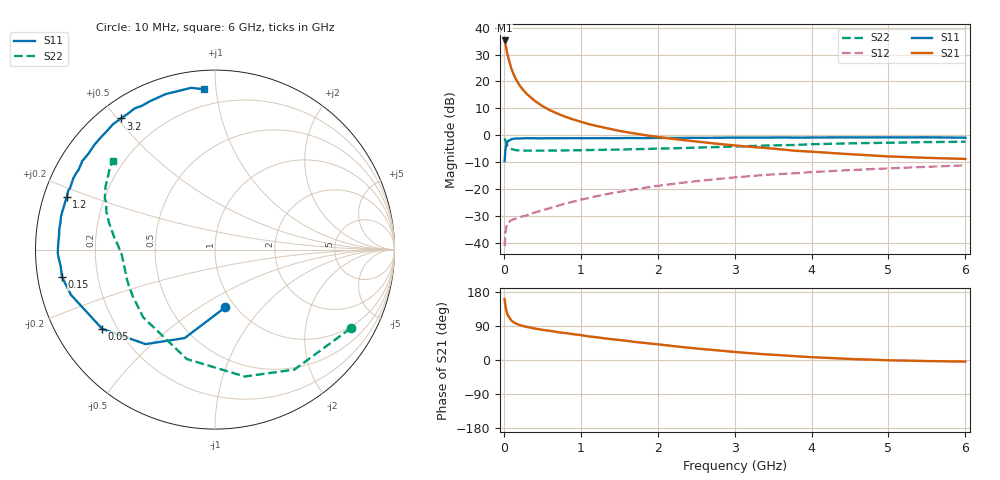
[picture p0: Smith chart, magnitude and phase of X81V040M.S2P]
! SIEMENS Small Signal Semiconductors
! BFP136W
! Si NPN RF Bipolar Junction Transistor in SOT343
! VCE = 1 V  IC = 40 mA
! Common Emitter S-Parameters:  September  1994
# GHz  S  MA  R  50
!  f  S11  S21  S12  S22
! GHz  MAG  ANG  MAG  ANG  MAG  ANG  MAG  ANG
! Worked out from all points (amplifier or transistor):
!   40 points, 10 MHz to 6 GHz, reference 50 ohm
!   highest |S21| = 35.2 dB at 10 MHz (marker M1)
!   |S21| within 3 dB of that: start of sweep to 32.17 MHz
!   unconditionally stable (mu >= 1): 616.7 MHz to 2.95 GHz; 3.767 GHz to 3.848 GHz; 5.876 GHz to end of sweep
!   at 200 MHz: K = 0.52, MSG = 24.6 dB, |S12| = -30.6 dB
!   at 1.5 GHz: K = 1.15, MAG = 9.0 dB, |S12| = -21.1 dB
!   at 6 GHz: K = 1.01, MAG = 0.5 dB, |S12| = -11.2 dB
!   S11 on the Smith chart (normalised r, x): 10 MHz: 0.90, -0.65; 50 MHz: 0.14, -0.31; 150 MHz: 0.07, -0.09; 1.2 GHz: 0.07, +0.17; 3.2 GHz: 0.07, +0.51; 6 GHz: 0.10, +0.93
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0.01  0.3272 -80.1  57.71 160.6  0.0086 69.3  0.874 -30.1
0.02  0.5209 -108.9  49.83 144.5  0.0151 55.6  0.8017 -56.5
0.03  0.6535 -126.3  42.35 132.8  0.0192 47.0  0.7262 -76.8
0.05  0.7679 -144.9  30.38 118.4  0.0234 34.8  0.6297 -104.4
0.1  0.8408 -162.5  16.84 103.5  0.0262 27.7  0.55 -136.7
0.15  0.866 -169.8  11.46 96.7  0.028 27.9  0.5267 -150.4
0.2  0.8647 -173.8  8.6 92.6  0.0295 30.1  0.52 -157.7
0.25  0.8722 -176.9  6.941 89.6  0.031 32.3  0.5177 -162.2
0.3  0.8766 -178.9  5.8 87.3  0.0323 34.6  0.5142 -165.4
0.4  0.8736 177.3  4.37 83.1  0.0364 39.3  0.5145 -169.4
0.5  0.8723 174.5  3.484 79.7  0.0397 43.3  0.5151 -172.1
0.6  0.8754 172.7  2.907 76.9  0.044 46.4  0.5169 -173.9
0.7  0.8741 170.0  2.506 73.6  0.0484 49.3  0.518 -175.1
0.9  0.8772 166.3  1.964 68.2  0.0578 52.2  0.5221 -177.5
1.1  0.8759 161.9  1.61 62.4  0.0676 54.1  0.5275 -179.1
1.2  0.8767 160.4  1.488 60.2  0.0728 54.6  0.531 -179.8
1.7  0.8829 151.2  1.074 47.8  0.0981 54.8  0.5475 176.3
2.2  0.8848 142.9  0.851 36.8  0.1239 52.4  0.569 172.4
3.2  0.8995 125.7  0.607 18.0  0.1725 44.1  0.6254 162.9
4.5  0.909 107.6  0.442 2.8  0.2237 32.2  0.7035 150.1
5.5  0.9111 98.4  0.378 -2.8  0.2577 24.2  0.7411 142.4
6  0.8959 94.1  0.361 -4.2  0.2742 19.8  0.7549 139.1
